//UDT 742.AWL
// ***************************************************************************


TYPE "ASTA_UDT"

STRUCT
	bType		: BYTE;			//ASTA-Typ
	bTA		: BYTE;			//Teilanlagenzuordnung
	boASTA_M	: BOOL;			//Anstoßmerker von Benutzer (ASTA_M-DB)
	boParamError	: BOOL;		//Fehler in Datensatz
	boParamErrorMsg	: BOOL;		//Meldung muß abgesetzt werden
	boError		: BOOL;		//Fehler beim Kettenstart (Typ1-4)
	boErrorMsg	: BOOL;			//Meldung muß abgesetzt werden
	bo5		: BOOL;
	boSendRecv  : BOOL;			//0=E7 mit Get/Put    1=E5 mit SendRecv
	boFP		: BOOL;			//pos. Flanke (gespeichert)
	bSrcSeq	: BYTE;			//Quell-Teilanlage
	bRemoteError: BYTE;			//Startfehler in remote PCU
	bRemoteOK	: BYTE;			//Start OK in remote PCU - nur Ebene4
	w		: WORD;			//Dummy
	u		: "XC_ASTA_UDT";
END_STRUCT

END_TYPE
